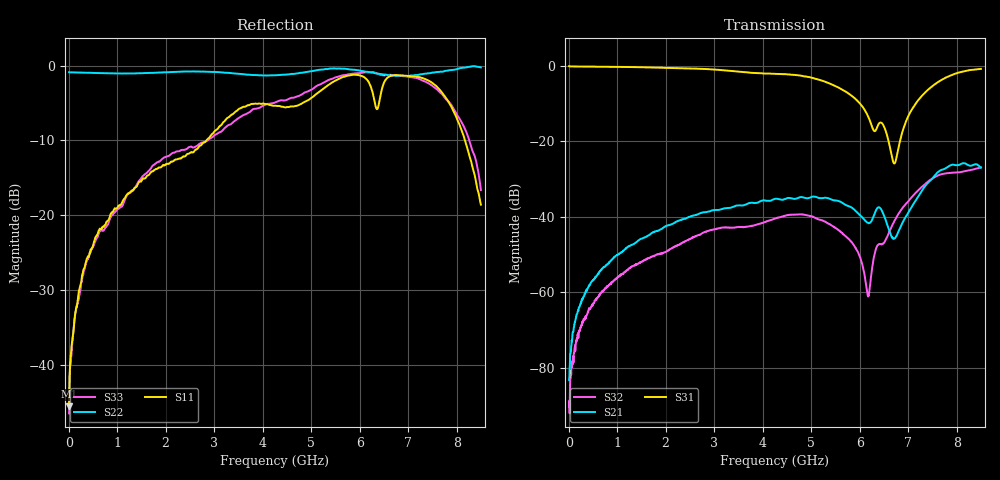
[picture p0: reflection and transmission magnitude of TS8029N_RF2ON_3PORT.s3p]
!Created with skrf (http://scikit-rf.org).
# GHz S RI R 50.0
!freq ReS11 ImS11 ReS12 ImS12 ReS13 ImS13
! ReS21 ImS21 ReS22 ImS22 ReS23 ImS23
! ReS31 ImS31 ReS32 ImS32 ReS33 ImS33
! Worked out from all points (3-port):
!   1601 points, 10 MHz to 8.5 GHz, reference 50 ohm
!   strongest paths, dB at 10 MHz, 2.132 GHz, 4.255 GHz, 6.378 GHz, 8.5 GHz:
!     S31: -0.1, -0.6, -2.1, -15.7, -0.8
!     S21: -83.3, -41.9, -35.3, -37.5, -27.0
!     S32: -90.4, -48.3, -40.5, -47.4, -26.9
!   lowest |S11| = -45.6 dB at 10 MHz (marker M1), VSWR 1.01, Z = 50.3 + j0.445 ohm
!   |S11| at or under -10 dB: start of sweep to 2.84 GHz; 8.171 GHz to end of sweep
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0.01  0.00284 0.00443  1.86e-05 5.31e-05  0.9922 -0.00969
      3.23e-05 6.05e-05  -0.9051 0.00334  2.16e-05 1.05e-05
      0.9919 -0.00966  2.09e-05 2.19e-05  0.00405 0.00243
0.30715  0.00782 -0.0426  4.47e-05 0.000895  0.9729 -0.1123
         2.54e-05 0.00087  -0.8942 0.0742  -7.61e-05 -0.000411
         0.9728 -0.1126  -7.37e-05 -0.000429  0.00296 -0.0415
0.965125  -0.0292 -0.1069  -0.000291 0.00298  0.9098 -0.3388
          -0.000309 0.003  -0.8543 0.244  -0.00128 -0.000763
          0.9095 -0.3384  -0.00129 -0.00075  -0.0235 -0.1029
4.255  -0.5401 0.023  0.0085 0.0151  -0.0687 -0.7831
       0.00842 0.0151  -0.3337 0.796  -0.000375 0.00944
       -0.0694 -0.7814  -0.000383 0.00945  -0.5666 -0.0159
5.576256  -0.5559 0.5983  0.0135 0.00883  -0.358 -0.3661
          0.0134 0.00884  -0.0318 0.9566  0.00499 0.00429
          -0.3576 -0.3657  0.00499 0.00428  -0.5637 0.6353
6.175863  -0.1318 0.776  0.00535 0.00632  -0.1892 -0.0988
          0.00538 0.0063  -0.00834 0.9089  -0.000122 0.000895
          -0.1889 -0.0988  -0.000144 0.000864  -0.4621 0.7758
6.3775  -0.2034 0.4819  0.00686 0.0113  -0.079 -0.1427
        0.00692 0.0113  0.0349 0.8844  -0.00335 0.00257
        -0.0788 -0.1429  -0.00338 0.00256  -0.2777 0.8367
6.7171  -0.1132 0.8571  0.00123 0.005  0.00479 -0.0507
        0.00125 0.00499  0.159 0.8425  -0.00805 0.00351
        0.00473 -0.0506  -0.0081 0.00348  0.1171 0.8571
7.210581  0.3786 0.7499  -0.00808 0.0168  0.2596 -0.2378
          -0.00806 0.0168  0.3774 0.7814  -0.0137 0.0178
          0.2595 -0.239  -0.0138 0.0178  0.5747 0.5817
8.5  0.0737 0.0916  0.0237 0.038  -0.2479 -0.8779
     0.0237 0.0381  0.5056 0.8337  0.0191 0.0407
     -0.2475 -0.8779  0.0192 0.0407  0.1448 0.0263
